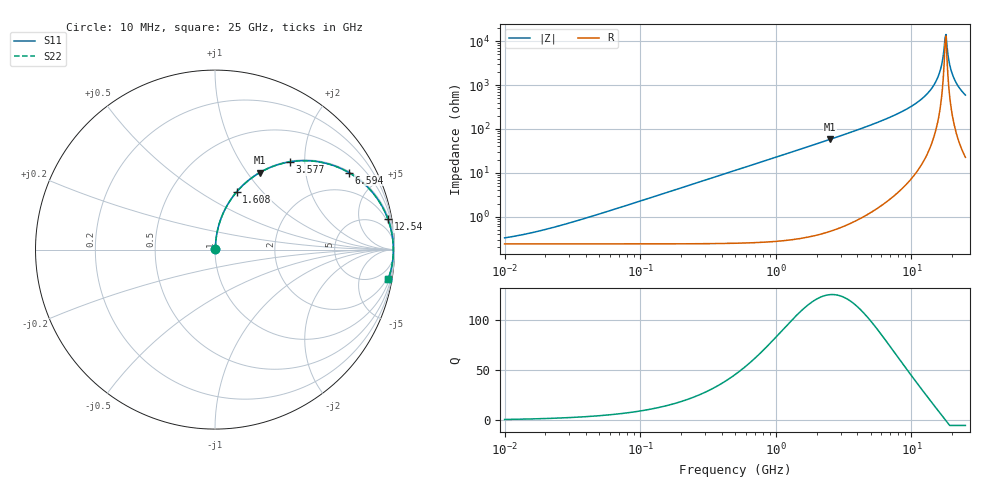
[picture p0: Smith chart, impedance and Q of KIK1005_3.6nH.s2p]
!version-3
!date-01.2023
!Series
# Hz S RI R 50
!Freq ReS11 ImS11 ReS21 ImS21 ReS12 ImS12 ReS22 ImS22
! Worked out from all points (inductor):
!   500 points, 10 MHz to 25 GHz, reference 50 ohm
!   read as one part in series: L = 3.6 nH near 31.91 MHz
!   highest Q = 125 at 2.494 GHz (marker M1), where L = 3.67 nH
!   self-resonance near 17.71 GHz
!   S11 on the Smith chart (normalised r, x): 10 MHz: 1.00, +0.00; 1.608 GHz: 1.01, +0.73; 3.577 GHz: 1.01, +1.69; 6.594 GHz: 1.04, +3.45; 12.54 GHz: 1, +11; 25 GHz: 1, -12
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1e7  0.0024 0.00225  0.9976 -0.00225  0.9976 -0.00225  0.0024 0.00225
3.732484e7  0.00246 0.0084  0.9975 -0.0084  0.9975 -0.0084  0.00246 0.0084
1.37147e8  0.00335 0.0308  0.9966 -0.0308  0.9966 -0.0308  0.00335 0.0308
5.039353e8  0.0152 0.1121  0.9848 -0.1121  0.9848 -0.1121  0.0152 0.1121
1.607969e9  0.1207 0.3213  0.8793 -0.3213  0.8793 -0.3213  0.1207 0.3213
1.851668e9  0.1541 0.3568  0.8459 -0.3568  0.8459 -0.3568  0.1541 0.3568
2.494271e9  0.2504 0.4293  0.7496 -0.4293  0.7496 -0.4293  0.2504 0.4293
3.577356e9  0.416 0.4887  0.584 -0.4887  0.584 -0.4887  0.416 0.4887
6.593752e9  0.7459 0.429  0.2541 -0.429  0.2541 -0.429  0.7459 0.429
6.803801e9  0.761 0.4199  0.239 -0.4199  0.239 -0.4199  0.761 0.4199
9.758208e9  0.903 0.2854  0.097 -0.2854  0.097 -0.2854  0.903 0.2854
1.254071e10  0.9629 0.1715  0.0371 -0.1715  0.0371 -0.1715  0.9629 0.1715
1.421668e10  0.9808 0.1116  0.0192 -0.1116  0.0192 -0.1116  0.9808 0.1116
1.561907e10  0.9891 0.0661  0.0109 -0.0661  0.0109 -0.0661  0.9891 0.0661
1.663003e10  0.9923 0.0356  0.00775 -0.0356  0.00775 -0.0356  0.9923 0.0356
1.743097e10  0.9934 0.0127  0.00662 -0.0127  0.00662 -0.0127  0.9934 0.0127
1.798625e10  0.9935 -0.00264  0.00645 0.00264  0.00645 0.00264  0.9935 -0.00264
1.827048e10  0.9935 -0.0103  0.00655 0.0103  0.00655 0.0103  0.9935 -0.0103
1.945306e10  0.9919 -0.0409  0.00811 0.0409  0.00811 0.0409  0.9919 -0.0409
2.038997e10  0.9895 -0.0638  0.0105 0.0638  0.0105 0.0638  0.9895 -0.0638
2.240132e10  0.9814 -0.1093  0.0186 0.1093  0.0186 0.1093  0.9814 -0.1093
2.5e10  0.9665 -0.1618  0.0335 0.1618  0.0335 0.1618  0.9665 -0.1618
